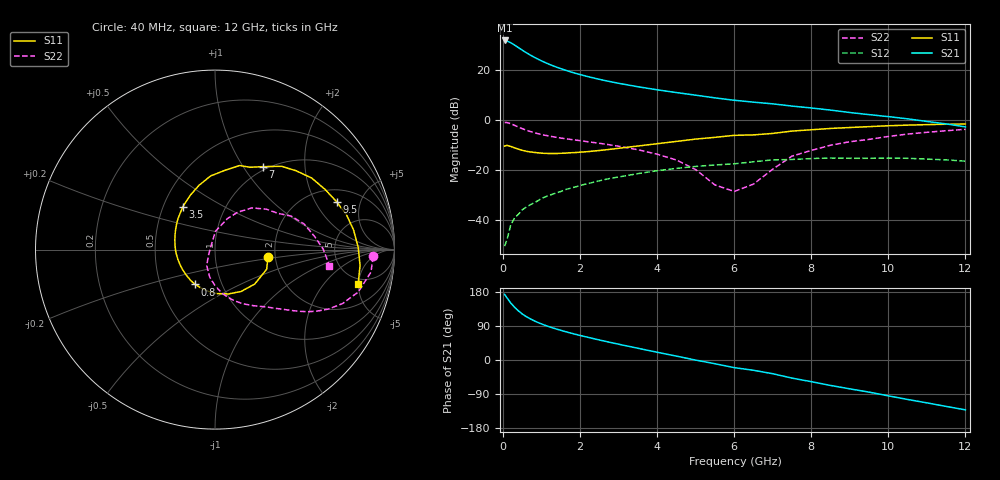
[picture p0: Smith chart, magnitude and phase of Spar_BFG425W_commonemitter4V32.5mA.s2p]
! Filename: 432bfg425.001
! BFG425W Field C1
! V1=8.380E-001V,V2=4.000E+000V, I1=4.223E-004A, I2=3.246E-002A
# GHz  S  MA  R 50
!  S11  S21  S12  S22
!Freq(GHz)  Mag  Ang  Mag  Ang  Mag  Ang  Mag  Ang
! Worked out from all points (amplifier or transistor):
!   44 points, 40 MHz to 12 GHz, reference 50 ohm
!   highest |S21| = 31.6 dB at 40 MHz (marker M1)
!   |S21| within 3 dB of that: start of sweep to 412.7 MHz
!   unconditionally stable (mu >= 1): start of sweep to 61.15 MHz; 1.05 GHz to end of sweep
!   at 700 MHz: K = 0.89, MSG = 29.9 dB, |S12| = -34.0 dB
!   at 2.4 GHz: K = 1.18, MAG = 18.0 dB, |S12| = -24.7 dB
!   at 12 GHz: K = 1.36, MAG = 3.3 dB, |S12| = -16.5 dB
!   S11 on the Smith chart (normalised r, x): 40 MHz: 1.83, -0.18; 800 MHz: 0.75, -0.31; 3.5 GHz: 0.63, +0.33; 7 GHz: 0.95, +1.23; 9.5 GHz: 2.68, +3.04; 12 GHz: 4.24, -4.93
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0.04  0.298 -8.4  38.15 173.0  0.003 41.9  0.882 -2.5
0.1  0.308 -20.8  37.18 164.2  0.004 66.8  0.878 -8.2
0.2  0.293 -40.9  34.37 150.3  0.008 68.0  0.832 -16.5
0.3  0.275 -58.0  30.8 139.1  0.011 67.3  0.772 -22.9
0.4  0.258 -73.5  27.41 129.5  0.013 65.9  0.714 -27.6
0.5  0.245 -87.8  24.39 121.2  0.016 64.4  0.663 -31.2
0.6  0.235 -99.6  21.81 114.6  0.018 63.5  0.62 -33.9
0.7  0.228 -109.8  19.65 109.0  0.02 62.6  0.584 -36.1
0.8  0.223 -119.6  17.82 103.8  0.022 62.0  0.554 -37.9
1  0.215 -135.7  14.91 95.1  0.027 61.0  0.507 -41.1
1.3  0.212 -154.6  11.88 84.4  0.033 59.4  0.457 -45.3
1.7  0.218 -174.8  9.288 72.6  0.042 56.5  0.41 -50.7
2.2  0.231 165.4  7.254 59.9  0.053 51.6  0.364 -58.1
2.8  0.258 145.8  5.712 46.1  0.068 44.7  0.313 -67.5
3.5  0.299 126.8  4.551 31.0  0.084 35.4  0.252 -79.7
4.5  0.369 104.0  3.483 10.2  0.107 20.6  0.157 -100.6
6.5  0.498 67.1  2.243 -27.1  0.145 -7.2  0.052 104.8
7  0.533 60.1  2.073 -36.2  0.158 -14.9  0.103 88.3
8.5  0.67 36.6  1.556 -67.2  0.172 -44.0  0.31 48.5
9.5  0.728 21.5  1.263 -84.8  0.17 -60.6  0.405 29.9
10.5  0.78 8.0  1.042 -104.2  0.17 -79.2  0.517 16.0
12  0.82 -13.4  0.72 -131.6  0.149 -109.0  0.644 -7.9
